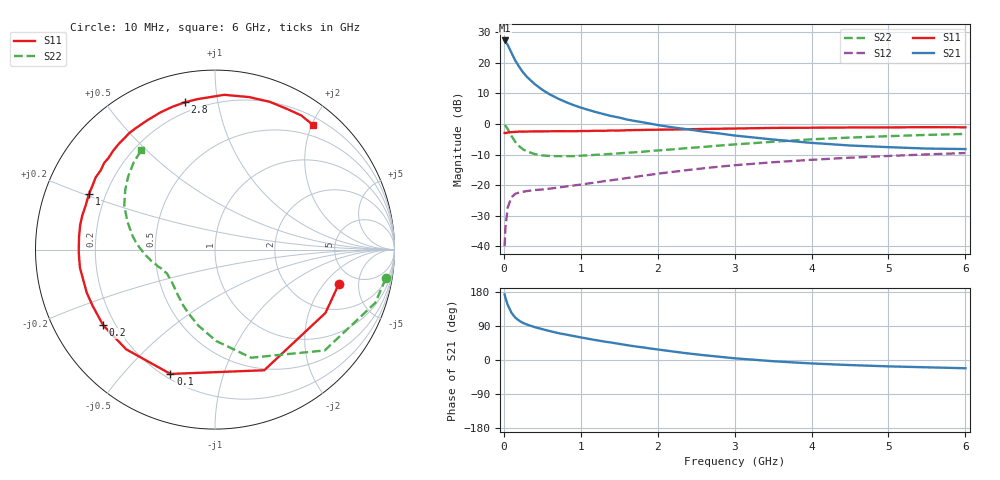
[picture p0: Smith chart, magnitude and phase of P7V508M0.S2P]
! SIEMENS Small Signal Semiconductors
! BFP196
! Si NPN RF Bipolar Junction Transistor in SOT143
! VCE = 0.5 V  IC = 8 mA
! Common Emitter S-Parameters:  May  1996
# GHz  S  MA  R  50
!  f  S11  S21  S12  S22
! GHz  MAG  ANG  MAG  ANG  MAG  ANG  MAG  ANG
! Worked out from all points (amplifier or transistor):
!   36 points, 10 MHz to 6 GHz, reference 50 ohm
!   highest |S21| = 27.3 dB at 10 MHz (marker M1)
!   |S21| within 3 dB of that: start of sweep to 79.52 MHz
!   unconditionally stable (mu >= 1): 869.4 MHz to end of sweep
!   at 250 MHz: K = 0.37, MSG = 19.5 dB, |S12| = -22.1 dB
!   at 1.4 GHz: K = 1.18, MAG = 7.9 dB, |S12| = -18.4 dB
!   at 6 GHz: K = 1.06, MAG = -0.8 dB, |S12| = -9.5 dB
!   S11 on the Smith chart (normalised r, x): 10 MHz: 3.65, -2.89; 100 MHz: 0.23, -0.68; 200 MHz: 0.15, -0.30; 1 GHz: 0.14, +0.21; 2.8 GHz: 0.15, +0.81; 6 GHz: 0.32, +2.03
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0.01  0.716 -15.6  23.19 173.2  0.0101 83.0  0.9644 -9.6
0.02  0.7094 -29.8  22.2 164.8  0.0198 76.8  0.9411 -18.4
0.05  0.726 -67.8  19.65 145.7  0.0432 58.3  0.8301 -42.6
0.1  0.7358 -109.7  14.5 124.4  0.0638 40.8  0.6351 -71.5
0.15  0.744 -131.7  10.82 111.8  0.0724 32.2  0.5089 -89.3
0.2  0.7523 -145.9  8.589 103.6  0.0762 27.5  0.4333 -102.4
0.25  0.7504 -155.4  6.976 97.8  0.0782 25.1  0.385 -112.5
0.3  0.7539 -161.5  5.893 93.6  0.0803 24.1  0.3579 -119.7
0.4  0.7593 -172.4  4.508 86.8  0.0834 23.4  0.3233 -130.6
0.5  0.7594 -178.9  3.625 81.4  0.0852 24.0  0.3073 -138.3
0.6  0.7607 174.9  3.035 76.2  0.0881 25.2  0.3002 -143.6
0.7  0.7636 169.6  2.62 71.3  0.0914 26.5  0.2983 -147.5
0.8  0.7634 165.4  2.3 67.4  0.095 27.4  0.2986 -150.5
1  0.7675 156.3  1.856 59.7  0.1025 29.9  0.3036 -155.5
1.1  0.7694 152.8  1.698 55.9  0.1069 31.1  0.3089 -157.5
1.6  0.7907 135.8  1.184 39.2  0.1311 34.0  0.3389 -165.5
2.2  0.8131 117.8  0.88 22.4  0.1656 33.0  0.3859 -174.9
2.8  0.8377 101.6  0.702 8.6  0.2011 28.9  0.4443 174.3
3.5  0.8639 86.6  0.558 -3.2  0.2376 21.7  0.513 162.2
4.5  0.878 69.8  0.446 -13.4  0.2821 11.0  0.6011 146.3
5.5  0.8886 57.3  0.397 -19.3  0.3191 0.3  0.6644 133.0
6  0.8834 51.6  0.39 -21.8  0.3357 -5.5  0.689 126.6
